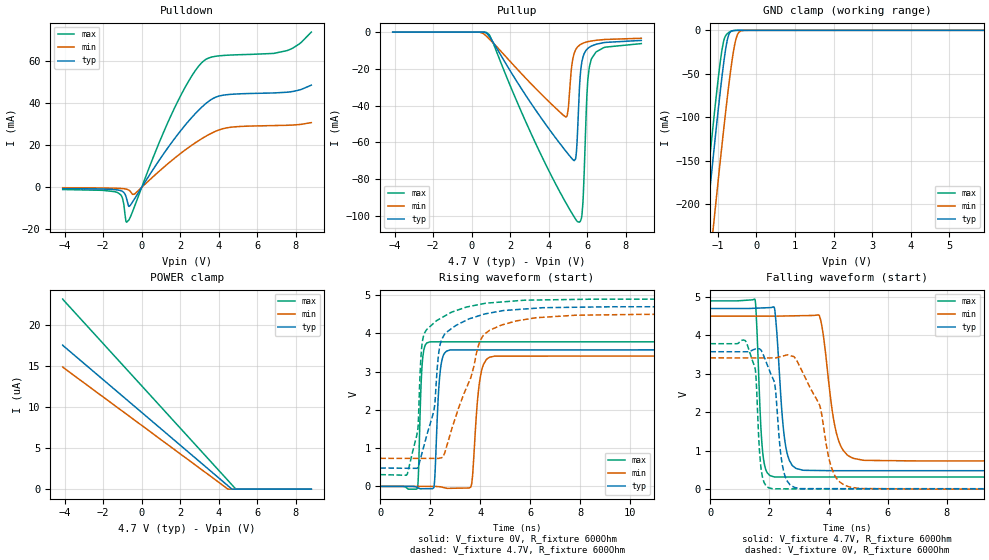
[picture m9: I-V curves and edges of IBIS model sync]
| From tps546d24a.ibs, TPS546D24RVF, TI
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|   sync Model
[Model]   sync
Model_type   I/O
Polarity   Non-Inverting
Enable   Active-High
Vinl = 0.8
Vinh = 1.35
Vmeas = 2.35
Vref = 0
Cref = 2pF
Rref = 100000
|   typ   min   max
C_comp   1.895pF   1.810pF   1.921pF
|C_comp_pull_up   1.643pF   1.548pF   1.744pF
|C_comp_pull_down   1.681pF   1.628pF   1.752pF
|  Where Nom  PVT is Nominal Process, 4.7V,  25C
|   Fast PVT is Strong Process,  4.9V,  -40C
|   Slow PVT is Weak Process,   4.5V,  150C
[Voltage Range]   4.7   4.5   4.9
|Junction Temperature
[Temperature Range]   25   150   -40
[Pullup Reference]   4.7   4.5   4.9
[Pulldown Reference]   0   0   0
[Power Clamp Reference]   4.7   4.5   4.9
[GND Clamp Reference]   0   0   0
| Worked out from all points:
|   slope of the pulldown table from 0 to 0.705 V, typ, clamps not added: 69.9 ohm
|   slope of the pullup table from 0 to 0.705 V, typ, clamps not added: 2.42 kohm
|   GND clamp passes 1 mA (typ) near -0.65 V on its own axis
|   falling waveform, V_fixture 4.7V, R_fixture 600Ohm: 20-80 % time 240ps typ, 392ps min, 156ps max; typ from 4.69 V to 0.479 V
|   rising waveform, V_fixture 0V, R_fixture 600Ohm: 20-80 % time 161ps typ, 238ps min, 113ps max; typ from 0 V to 3.57 V
|   rising waveform, V_fixture 4.7V, R_fixture 600Ohm: 20-80 % time 617ps typ, 1.11ns min, 338ps max; typ from 0.479 V to 4.69 V
|   falling waveform, V_fixture 0V, R_fixture 600Ohm: 20-80 % time 292ps typ, 734ps min, 155ps max; typ from 3.57 V to 0 V
[Pulldown]
|   Voltage   I(typ)   I(min)   I(max)
-4.1V     -553.3uA   -191.1uA   -1.04mA
-1.236V   -1.267mA   -459.3uA   -2.551mA
-991.1mV  -1.98mA    -596.6uA   -5.399mA
-784.7mV  -5.424mA   -895.9uA   -16.56mA
-681.5mV  -8.966mA   -1.268mA   -15.68mA
-604.1mV  -8.673mA   -1.827mA   -14.39mA
-371.9mV  -5.447mA   -3.165mA   -9.064mA
1.666V    22.68mA    13.55mA    37mA
3.111V    38.05mA    23.09mA    59.2mA
4.195V    43.73mA    27.82mA    62.61mA
7.549V    45.18mA    29.48mA    64.97mA
8.8V      48.55mA    30.75mA    73.75mA
[GND Clamp]
|   Voltage   I(typ)   I(min)   I(max)
-4.1V     -1.516A    -1.586A    -1.487A
-1.417V   -274.6mA   -356.5mA   -236.8mA
-1.275V   -211.7mA   -293.9mA   -173.6mA
-1.159V   -161mA     -243.2mA   -123.1mA
-1.081V   -127.9mA   -209.8mA   -90.42mA
-952.4mV  -74.94mA   -155.2mA   -40.34mA
-862.1mV  -41.13mA   -118.2mA   -14.25mA
-758.9mV  -11.34mA   -77.77mA   -3.876mA
-655.7mV  -1.062mA   -41.33mA   -972.9uA
-500.9mV  -29.19uA   -5.608mA   -29.82uA
-320.3mV  -695.3nA   -63.7uA    -811.2nA
8.8V      0A         0A         0A
[Pullup]
|   Voltage   I(typ)   I(min)   I(max)
-4.1V     705fA      -189.7pA   1.158pA
905.2mV   -2.271mA   -3.656mA   -1.34mA
4.878V    -64.67mA   -46.13mA   -92.71mA
5.007V    -66.35mA   -41.89mA   -95.07mA
5.162V    -68.34mA   -21.05mA   -97.83mA
5.304V    -69.83mA   -12.02mA   -100.3mA
5.433V    -65.12mA   -8.914mA   -102.4mA
5.588V    -30.72mA   -7.141mA   -103.4mA
5.769V    -13.74mA   -6.06mA    -92.99mA
5.975V    -9.4mA     -5.349mA   -34.68mA
6.194V    -7.673mA   -4.866mA   -15.11mA
8.8V      -4.538mA   -3.348mA   -6.264mA
[POWER Clamp]
|   Voltage   I(typ)   I(min)   I(max)
-4.1V     17.58uA    14.91uA    23.2uA
4.466V    431.3nA    15.83nA    1.085uA
4.672V    16.85nA    0A         551.8nA
4.878V    0A         0A         17.9nA
8.8V      0A         0A         0A
[Ramp]
R_load = 600
|   typ   min   max
dV/dt_r   2.14282/1.60795e-10   2.04663/2.37639e-10   2.26793/1.13163e-10
dV/dt_f   2.52902/2.39541e-10   2.25739/3.90759e-10   2.75104/1.56026e-10
[Falling Waveform]
V_fixture = 4.7V
V_fixture_min = 4.5V
V_fixture_max = 4.9V
R_fixture = 600Ohm
C_fixture = 0F
|   Time   V(typ)   V(min)   V(max)
0s        4.694V     4.495V     4.892V
1.512ns   4.701V     4.495V     4.93V
1.784ns   4.71V      4.495V     884.2mV
2.173ns   4.695V     4.495V     316.9mV
2.566ns   1.05V      4.501V     316.8mV
3.132ns   492.9mV    4.509V     316.7mV
3.693ns   484.3mV    4.501V     316.6mV
4.334ns   479.6mV    1.275V     316.5mV
5.165ns   479.6mV    752.3mV    316.3mV
50ns      479.3mV    733mV      307.4mV
[Rising Waveform]
V_fixture = 0V
V_fixture_min = 0V
V_fixture_max = 0V
R_fixture = 600Ohm
C_fixture = 0F
|   Time   V(typ)   V(min)   V(max)
0s        4.652uV    24.31uV    2.367uV
1.488ns   -29.57mV   -28.68uV   -47.82mV
1.686ns   -62.69mV   -35.73uV   3.264V
1.985ns   -60.35mV   -46.37uV   3.775V
2.419ns   3.109V     -12.13mV   3.775V
2.804ns   3.564V     -50.11mV   3.775V
3.623ns   3.564V     -19.19mV   3.775V
4.028ns   3.564V     2.941V     3.775V
4.582ns   3.564V     3.403V     3.775V
50ns      3.571V     3.411V     3.78V
[Rising Waveform]
V_fixture = 4.7V
V_fixture_min = 4.5V
V_fixture_max = 4.9V
R_fixture = 600Ohm
C_fixture = 0F
|   Time   V(typ)   V(min)   V(max)
0s        479.3mV    733mV      307.4mV
1.047ns   473.5mV    731.6mV    290.8mV
1.516ns   494.2mV    731mV      1.588V
1.622ns   751.9mV    730.8mV    3.323V
1.716ns   980.5mV    730.7mV    3.889V
2.155ns   2.018V     730.1mV    4.272V
2.344ns   3.507V     732.8mV    4.363V
2.499ns   3.884V     756.1mV    4.42V
4.226ns   4.509V     4.003V     4.785V
50ns      4.694V     4.495V     4.892V
[Falling Waveform]
|Gnd
V_fixture = 0V
V_fixture_min = 0V
V_fixture_max = 0V
R_fixture = 600Ohm
C_fixture = 0F
|   Time   V(typ)   V(min)   V(max)
0s        3.571V     3.411V     3.78V
1.216ns   3.57V      3.41V      3.822V
1.525ns   3.644V     3.41V      3.093V
1.753ns   3.56V      3.41V      361.1mV
2.124ns   2.864V     3.41V      8.273mV
2.698ns   112.1mV    3.472V     8.174mV
3.701ns   13.25mV    2.176V     8.001mV
4.201ns   13.11mV    369.4mV    7.914mV
5.012ns   12.88mV    20.58mV    7.774mV
50ns      4.783uV    24.57uV    2.434uV
